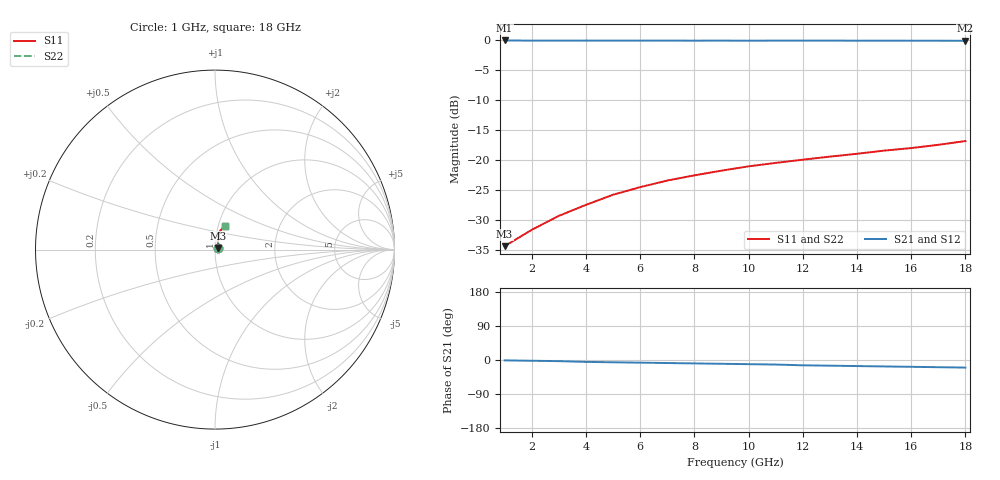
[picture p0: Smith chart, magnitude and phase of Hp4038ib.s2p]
!HPND-4038 beam lead PIN diode
!Series configuration S-parameters If= 5 mA.  Last updated 10/3/97
# mhz s ma r 50
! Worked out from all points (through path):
!   18 points, 1 GHz to 18 GHz, reference 50 ohm
!   highest |S21| = -0.11 dB at 1 GHz (marker M1); lowest = -0.2 dB at 18 GHz (marker M2)
!   group delay of S21, straight-line fit = 3.13 ps
!   lowest |S11| = -34.4 dB at 1 GHz (marker M3), VSWR 1.04, Z = 51.7 + j0.923 ohm
!   |S11| at or under -10 dB: start of sweep to end of sweep
!   |S22| runs from -34.4 to -16.9 dB; largest |S21 - S12| = 0
1000  0.019 28.0  0.987 -1.0  0.987 -1.0  0.019 28.0
2000  0.026 50.0  0.984 -2.0  0.984 -2.0  0.026 50.0
3000  0.034 61.0  0.985 -3.0  0.985 -3.0  0.034 61.0
4000  0.042 67.0  0.985 -5.0  0.985 -5.0  0.042 67.0
5000  0.051 72.0  0.984 -6.0  0.984 -6.0  0.051 72.0
6000  0.059 74.0  0.984 -7.0  0.984 -7.0  0.059 74.0
7000  0.067 76.0  0.984 -8.0  0.984 -8.0  0.067 76.0
8000  0.074 76.0  0.983 -9.0  0.983 -9.0  0.074 76.0
9000  0.081 77.0  0.984 -10.0  0.984 -10.0  0.081 77.0
10000  0.088 77.0  0.982 -11.0  0.982 -11.0  0.088 77.0
11000  0.094 77.0  0.984 -12.0  0.984 -12.0  0.094 77.0
12000  0.1 76.0  0.984 -14.0  0.984 -14.0  0.1 76.0
13000  0.106 75.0  0.985 -15.0  0.985 -15.0  0.106 75.0
14000  0.112 74.0  0.982 -16.0  0.982 -16.0  0.112 74.0
15000  0.119 72.0  0.983 -17.0  0.983 -17.0  0.119 72.0
16000  0.125 71.0  0.982 -18.0  0.982 -18.0  0.125 71.0
17000  0.133 68.0  0.982 -19.0  0.982 -19.0  0.133 68.0
18000  0.143 66.0  0.98 -20.0  0.98 -20.0  0.143 66.0
